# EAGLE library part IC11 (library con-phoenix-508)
PHOENIX
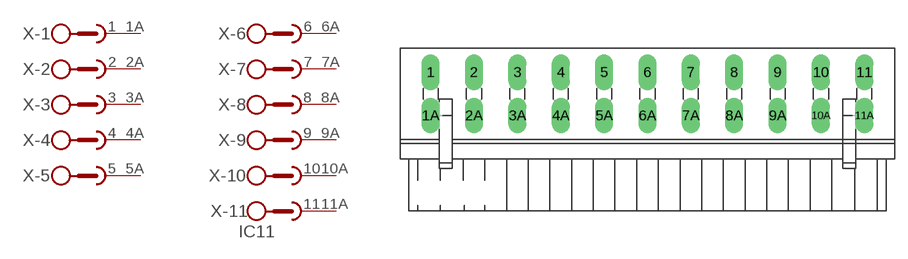
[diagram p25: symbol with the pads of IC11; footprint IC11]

Designator prefix X; gates -1=SKB2 -2=SKB2 -3=SKB2 -4=SKB2 -5=SKB2 -6=SKB2 -7=SKB2 -8=SKB2 -9=SKB2 -10=SKB2 -11=SKB2V

## IC11 (OC_FARNELL: unknown; OC_NEWARK: unknown)  [IC11]
1  -1:1  pas
1A  -1:2  pas
2  -2:1  pas
2A  -2:2  pas
3  -3:1  pas
3A  -3:2  pas
4  -4:1  pas
4A  -4:2  pas
5  -5:1  pas
5A  -5:2  pas
6  -6:1  pas
6A  -6:2  pas
7  -7:1  pas
7A  -7:2  pas
8  -8:1  pas
8A  -8:2  pas
9  -9:1  pas
9A  -9:2  pas
10  -10:1  pas
10A  -10:2  pas
11  -11:1  pas
11A  -11:2  pas

## Footprint IC11 (pad centres in mm)
PHOENIX
drill 1.397 long: 1 -25.4,2.54; 1A -25.4,-2.54; 2 -20.32,2.54; 2A -20.32,-2.54; 3 -15.24,2.54; 3A -15.24,-2.54; 4 -10.16,2.54; 4A -10.16,-2.54; 5 -5.08,2.54; 5A -5.08,-2.54; 6 0,2.54; 6A 0,-2.54; 7 5.08,2.54; 7A 5.08,-2.54; 8 10.16,2.54; 8A 10.16,-2.54; 9 15.24,2.54; 9A 15.24,-2.54; 10 20.32,2.54; 10A 20.32,-2.54; 11 25.4,2.54; 11A 25.4,-2.54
